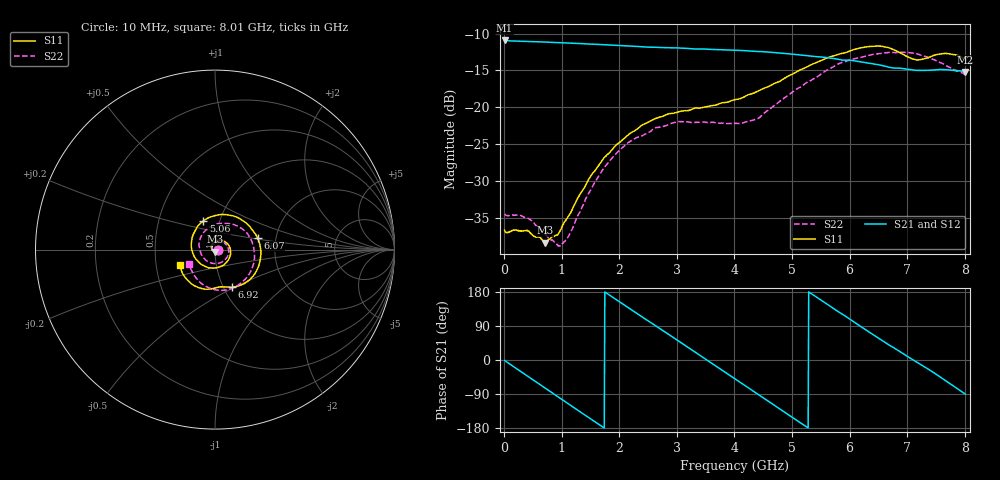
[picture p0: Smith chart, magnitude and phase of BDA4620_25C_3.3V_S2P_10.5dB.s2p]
!Agilent Technologies,E5071B,MY42404982,A.09.10
!Date: Wed May 06 08:50:39 2026
!Data & Calibration Information:
!Freq	S11:SOLT2(ON)	S21:SOLT2(ON)	S12:SOLT2(ON)	S22:SOLT2(ON)
# Hz S RI R 50
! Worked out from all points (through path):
!   801 points, 10 MHz to 8.01 GHz, reference 50 ohm
!   highest |S21| = -10.93 dB at 10 MHz (marker M1); lowest = -15.2 dB at 8.01 GHz (marker M2)
!   group delay of S21, straight-line fit = 281 ps
!   lowest |S11| = -38.3 dB at 710 MHz (marker M3), VSWR 1.02, Z = 49.9 - j1.2 ohm
!   |S11| at or under -10 dB: start of sweep to end of sweep
!   |S22| runs from -38.8 to -12.5 dB; largest |S21 - S12| = 0.0013
!   S11 on the Smith chart (normalised r, x): 10 MHz: 1.03, -0.00; 5.06 GHz: 0.84, +0.27; 6.07 GHz: 1.60, +0.22; 6.92 GHz: 1.09, -0.48; 8.01 GHz: 0.67, -0.12
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1e7  0.0146 -0.00102  0.2839 -0.00608  0.2843 -0.00619  0.0188 -0.00113
4.1e8  0.0104 -0.0102  0.2049 -0.1902  0.2049 -0.1907  0.0142 -0.0106
7.1e8  -0.000987 -0.0121  0.0767 -0.2661  0.0766 -0.2666  0.00329 -0.0135
9.9e8  -0.014 -0.0051  -0.0603 -0.2672  -0.0606 -0.2678  -0.00913 -0.00717
1.35e9  -0.0203 0.0177  -0.2061 -0.1749  -0.2064 -0.175  -0.0162 0.0131
1.94e9  0.0171 0.0525  -0.2478 0.0892  -0.2482 0.0895  0.0129 0.0466
2.32e9  0.0581 0.0419  -0.1351 0.2207  -0.1355 0.221  0.0479 0.0405
2.68e9  0.0853 0.00336  0.0204 0.2541  0.0207 0.2543  0.0718 0.0136
3e9  0.0807 -0.045  0.1517 0.2021  0.1521 0.2022  0.0762 -0.0233
3.39e9  0.0374 -0.0915  0.2417 0.059  0.2421 0.0587  0.0458 -0.0645
4.01e9  -0.0782 -0.0811  0.1584 -0.1855  0.1586 -0.1857  -0.0469 -0.0622
4.51e9  -0.1324 0.0225  -0.0439 -0.2342  -0.0442 -0.2345  -0.0887 0.0203
5.06e9  -0.0655 0.1591  -0.2099 -0.0896  -0.2105 -0.0894  -0.0247 0.1288
5.35e9  0.023 0.1945  -0.2207 0.0245  -0.2208 0.0246  0.0482 0.146
5.67e9  0.1345 0.1743  -0.168 0.1352  -0.1682 0.1356  0.1336 0.1264
6.07e9  0.2373 0.0649  -0.0393 0.2031  -0.0393 0.2035  0.2104 0.0311
6.38e9  0.2504 -0.0665  0.0689 0.1855  0.0689 0.1857  0.2179 -0.0648
6.68e9  0.1794 -0.179  0.1431 0.1203  0.1437 0.1204  0.1784 -0.1537
6.92e9  0.0935 -0.2097  0.1748 0.0551  0.1751 0.0551  0.1191 -0.2039
7.19e9  0.0285 -0.2075  0.1761 -0.0241  0.1767 -0.0243  0.0288 -0.2274
7.57e9  -0.0814 -0.2149  0.1286 -0.1268  0.1288 -0.1269  -0.0809 -0.1843
8.01e9  -0.193 -0.0847  -0.000134 -0.1739  4.52e-05 -0.1744  -0.1464 -0.079
